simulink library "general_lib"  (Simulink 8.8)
settings: Solver=ode45  StartTime=0.0  StopTime=10.0  RelTol=1e-3  EnableMultiTasking=on
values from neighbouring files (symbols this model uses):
  transmission = class_transmission_data    [class_test_data.m]
undefined symbols (not defined in the file or in its folder): AxisNumber, BreakpointData, BreakpointsForDimension1, BreakpointsForDimension2, BreakpointsForDimension3, DelayTimeSecs, down_time, ExtrapolateAbove, ExtrapolateBelow, InitialCondition, InitialValue, LookupStructure, MaximumIndicesForEachDimension, MultiplyPosInputs, Normalize, NumPhases, struct_var, Table, test_mat, up_time, UpperSaturationLimit, VerboseLevel, VerboseSignal
libraries: general_lib x5, simulink x3

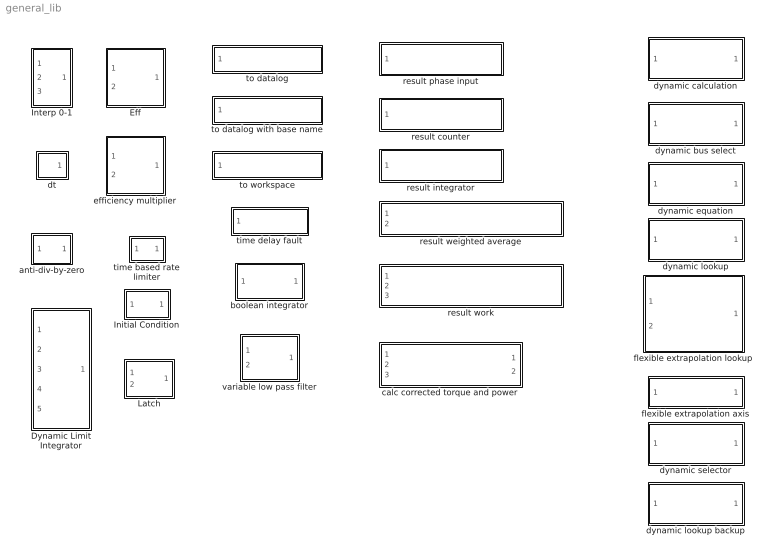
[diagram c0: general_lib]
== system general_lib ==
  Dynamic Limit Integrator : Subsystem
  Eff : Subsystem
  Initial Condition : Subsystem
  Interp 0-1 : Subsystem
  Latch : Subsystem
  anti-div-by-zero : Subsystem
  boolean integrator : Subsystem
  calc corrected torque and power : Subsystem
  dt : Subsystem
  dynamic bus select : Subsystem
  dynamic calculation : Subsystem
  dynamic equation : Subsystem
  dynamic lookup : Subsystem
  dynamic lookup backup : Subsystem  Commented=on
  dynamic selector : Subsystem  BlockChoice=dynamic equation
  efficiency multiplier : Subsystem
  flexible extrapolation axis : Subsystem
  flexible extrapolation lookup : Subsystem
  result counter : Subsystem
  result integrator : Subsystem
  result phase input : Subsystem
  result weighted average : Subsystem
  result work : Subsystem
  time based rate limiter : Subsystem
  time delay fault : Subsystem
  to datalog : Subsystem
  to datalog with base name : Subsystem
  to workspace : Subsystem
  variable low pass filter : Subsystem

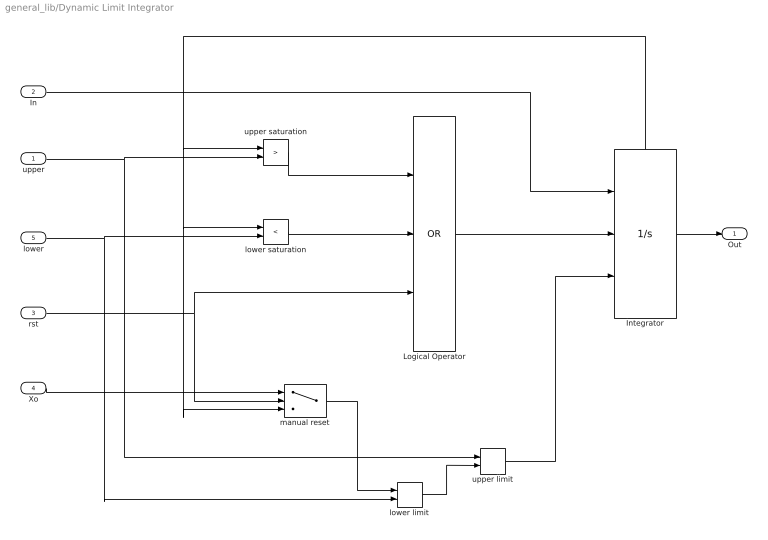
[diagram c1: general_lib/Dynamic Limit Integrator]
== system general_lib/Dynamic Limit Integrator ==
  upper : Inport
  In : Inport  Port=2
  rst : Inport  Port=3
  Xo : Inport  Port=4
  lower : Inport  Port=5
  Integrator : Integrator  ExternalReset=level  InitialConditionSource=external  ShowStatePort=on
  Logical Operator : Logic  Operator=OR  Inputs=3  AllPortsSameDT=off  OutDataTypeStr=boolean
  lower limit : MinMax  Function=max  Inputs=2  ZeroCross=off
  lower saturation : RelationalOperator  Operator=<  OutDataTypeStr=boolean
  manual reset : Switch  Criteria=u2 ~= 0
  upper limit : MinMax  Inputs=2
  upper saturation : RelationalOperator  Operator=>  OutDataTypeStr=boolean
  Out : Outport
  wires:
  Integrator/State -> manual reset/3, lower saturation/1, upper saturation/1
  Integrator/1 -> Out/1
  lower limit/1 -> upper limit/2
  Xo/1 -> manual reset/1
  rst/1 -> manual reset/2, Logical Operator/3
  upper saturation/1 -> Logical Operator/1
  lower saturation/1 -> Logical Operator/2
  Logical Operator/1 -> Integrator/2
  In/1 -> Integrator/1
  lower/1 -> lower limit/2, lower saturation/2
  upper limit/1 -> Integrator/3
  upper/1 -> upper saturation/2, upper limit/1
  manual reset/1 -> lower limit/1

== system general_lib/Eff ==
  Efficiency : Inport
  Input : Inport  Port=2
  Math Function : Math  Operator=reciprocal
  Product1 : Product
  Switch : Switch  ZeroCross=off
  Output : Outport
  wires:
  Switch/1 -> Product1/1
  Efficiency/1 -> Math Function/1, Switch/1
  Input/1 -> Switch/2, Product1/2
  Product1/1 -> Output/1
  Math Function/1 -> Switch/3

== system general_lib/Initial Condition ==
  In : Inport
  Constant2 : Constant
  IC Switch : Switch  Criteria=u2 ~= 0
  IC Value : Constant  Value=InitialValue
  Memory : Memory
  Out : Outport
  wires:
  IC Switch/1 -> Out/1
  In/1 -> IC Switch/1
  IC Value/1 -> IC Switch/3
  Memory/1 -> IC Switch/2
  Constant2/1 -> Memory/1

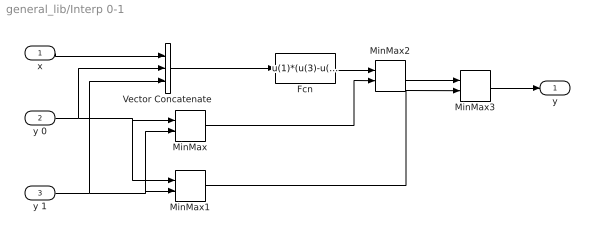
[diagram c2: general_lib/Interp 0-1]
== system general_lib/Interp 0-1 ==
  x : Inport
  y 0 : Inport  Port=2
  y 1 : Inport  Port=3
  Fcn : Fcn  Expr=u(1)*(u(3)-u(2)) + u(2)
  MinMax : MinMax  Inputs=2  ZeroCross=off
  MinMax1 : MinMax  Function=max  Inputs=2  ZeroCross=off
  MinMax2 : MinMax  Function=max  Inputs=2  ZeroCross=off
  MinMax3 : MinMax  Inputs=2  ZeroCross=off
  Vector Concatenate : Concatenate  NumInputs=3
  y : Outport
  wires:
  y 0/1 -> Vector Concatenate/2, MinMax1/1, MinMax/1
  Vector Concatenate/1 -> Fcn/1
  y 1/1 -> Vector Concatenate/3, MinMax/2, MinMax1/2
  MinMax3/1 -> y/1
  x/1 -> Vector Concatenate/1
  MinMax/1 -> MinMax2/2
  MinMax1/1 -> MinMax3/2
  MinMax2/1 -> MinMax3/1
  Fcn/1 -> MinMax2/1

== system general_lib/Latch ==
  On : Inport  PortDimensions=1
  Off : Inport  Port=2  PortDimensions=1
  Combinatorial  Logic : CombinatorialLogic  TruthTable=[0;1;0;0;1;1;(tb==2);(tb>=2)]
  Memory2 : Memory  X0=InitialCondition
  Mux : Mux  Inputs=3
  State : Outport  PortDimensions=1
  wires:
  Combinatorial  Logic/1 -> Memory2/1, State/1
  Mux/1 -> Combinatorial  Logic/1
  Memory2/1 -> Mux/3
  On/1 -> Mux/1
  Off/1 -> Mux/2

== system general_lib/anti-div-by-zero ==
  note: force sign(0) = 1, not 0!
  In : Inport
  Abs : Abs  ZeroCross=off
  Constant : Constant  Value=eps
  MinMax : MinMax  Function=max  Inputs=2  ZeroCross=off
  Product2 : Product
  Relay : Relay  OnSwitchValue=-eps  OffSwitchValue=-eps  OffOutputValue=-1  ZeroCross=off
  Out : Outport
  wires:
  Product2/1 -> Out/1
  In/1 -> Relay/1, Abs/1
  Abs/1 -> MinMax/1
  MinMax/1 -> Product2/1
  Constant/1 -> MinMax/2
  Relay/1 -> Product2/2

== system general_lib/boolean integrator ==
  bool : Inport
  Constant : Constant  Value=Normalize
  Data Type Conversion2 : DataTypeConversion  OutDataTypeStr=double
  Integrator1 : Integrator  ExternalReset=falling  LimitOutput=on  UpperSaturationLimit=UpperSaturationLimit  LowerSaturationLimit=0
  Switch : Switch  Criteria=u2 > Threshold
  normalize : Gain  Gain=1/UpperSaturationLimit
  out : Outport
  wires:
  Data Type Conversion2/1 -> Integrator1/2, Integrator1/1
  bool/1 -> Data Type Conversion2/1
  Constant/1 -> Switch/2
  Integrator1/1 -> normalize/1, Switch/3
  normalize/1 -> Switch/1
  Switch/1 -> out/1

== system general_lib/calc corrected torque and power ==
  trq_Nm : Inport
  spd_radps : Inport  Port=2
  upstream_iner_kgm2 : Inport  Port=3
  Derivative : Derivative  CoefficientInTFapproximation=1e6
  Product1 : Product
  Product2 : Product
  Subtract : Sum  Inputs=+-
  corr_trq_Nm : Outport
  corr_pwr_W : Outport  Port=2
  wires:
  trq_Nm/1 -> Subtract/1
  Subtract/1 -> Product2/1, corr_trq_Nm/1
  upstream_iner_kgm2/1 -> Product1/2
  spd_radps/1 -> Product2/2, Derivative/1
  Derivative/1 -> Product1/1
  Product1/1 -> Subtract/2
  Product2/1 -> corr_pwr_W/1

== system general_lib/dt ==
  Clock : Clock
  Memory1 : Memory
  Sum : Sum  Inputs=|-+
  dt : Outport
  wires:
  Sum/1 -> dt/1
  Memory1/1 -> Sum/1
  Clock/1 -> Memory1/1, Sum/2

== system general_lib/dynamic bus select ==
  bus : Inport
  Bus Selector : BusSelector  OutputSignals=signal1,bus.signal2  OutputAsBus=on
  Reshape : Reshape
  out : Outport
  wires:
  Reshape/1 -> out/1
  bus/1 -> Bus Selector/1
  Bus Selector/1 -> Reshape/1

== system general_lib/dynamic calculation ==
  bus : Inport
  dynamic selector : Subsystem  BlockChoice=dynamic equation
  out : Outport
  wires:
  bus/1 -> dynamic selector/1(bus)
  dynamic selector/1(out) -> out/1

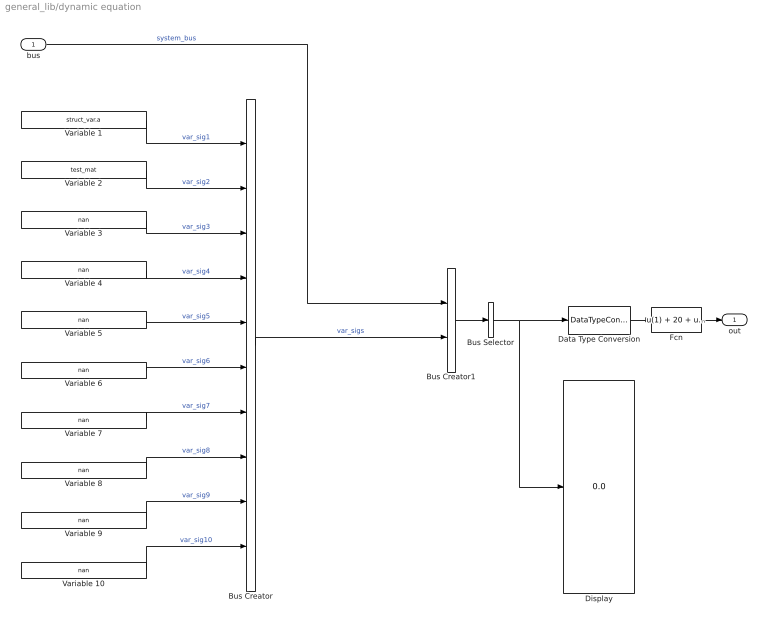
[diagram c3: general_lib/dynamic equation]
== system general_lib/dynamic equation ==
  bus : Inport
  Bus Creator : BusCreator  Inputs=10
  Bus Creator1 : BusCreator  Inputs=2
  Bus Selector : BusSelector  OutputSignals=sig_1,var_sigs.var_sig1,var_sigs.var_sig2  OutputAsBus=on
  Data Type Conversion : DataTypeConversion  OutDataTypeStr=double
  Display : Display
  Fcn : Fcn  Expr=u(1) + 20 + u(3) + u(2)
  Variable 1 : Constant  Value=struct_var.a
  Variable {3..10} (8 alike) : Constant  Value=nan
  Variable 2 : Constant  Value=test_mat
  out : Outport
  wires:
  Variable 10/1 -> Bus Creator/10  "var_sig10"
  Variable 9/1 -> Bus Creator/9  "var_sig9"
  Variable 8/1 -> Bus Creator/8  "var_sig8"
  Variable 7/1 -> Bus Creator/7  "var_sig7"
  Variable 6/1 -> Bus Creator/6  "var_sig6"
  Variable 5/1 -> Bus Creator/5  "var_sig5"
  Variable 4/1 -> Bus Creator/4  "var_sig4"
  Variable 3/1 -> Bus Creator/3  "var_sig3"
  Variable 2/1 -> Bus Creator/2  "var_sig2"
  Variable 1/1 -> Bus Creator/1  "var_sig1"
  Bus Creator/1 -> Bus Creator1/2  "var_sigs"
  bus/1 -> Bus Creator1/1  "system_bus"
  Fcn/1 -> out/1
  Bus Creator1/1 -> Bus Selector/1
  Bus Selector/1 -> Display/1, Data Type Conversion/1
  Data Type Conversion/1 -> Fcn/1

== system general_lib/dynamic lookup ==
  bus : Inport
  Bus Selector : BusSelector  OutputSignals=gb.gb_cmd_gear,gb_spd_in_radps,ctrl.gb_line_press_bar
  Lookup : Lookup_n-D  NumberOfTableDimensions=10  BreakpointsForDimension1=LookupStructure.axis_1.breakpoints  BreakpointsForDimension2=LookupStructure.axis_2.breakpoints  BreakpointsForDimension3=LookupStructure.axis_3.breakpoints  BreakpointsForDimension4=LookupStructure.axis_4.breakpoints  BreakpointsForDimension5=LookupStructure.axis_5.breakpoints  BreakpointsForDimension6=LookupStructure.axis_6.breakpoints  BreakpointsForDimension7=LookupStructure.axis_7.breakpoints  BreakpointsForDimension8=LookupStructure.axis_8.breakpoints  BreakpointsForDimension9=LookupStructure.axis_9.breakpoints  BreakpointsForDimension10=LookupStructure.axis_10.breakpoints  IndexSearchMethod=Linear search  BeginIndexSearchUsingPreviousIndexResult=on  Table=LookupStructure.table  DiagnosticForOutOfRangeInput=Warning  InternalRulePriority=Speed  RndMeth=Simplest  SupportTunableTableSize=on  MaximumIndicesForEachDimension=LookupStructure.table_size
  out : Outport
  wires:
  Lookup/1 -> out/1
  bus/1 -> Bus Selector/1

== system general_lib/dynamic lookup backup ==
  bus : Inport
  Bus Selector : BusSelector  OutputSignals=gb.gb_cmd_gear,gb_spd_in_radps,ctrl.gb_line_press_bar
  Lookup : Lookup_n-D  NumberOfTableDimensions=10  BreakpointsForDimension1=LookupStructure.axis_1.breakpoints  BreakpointsForDimension2=LookupStructure.axis_2.breakpoints  BreakpointsForDimension3=LookupStructure.axis_3.breakpoints  BreakpointsForDimension4=LookupStructure.axis_4.breakpoints  BreakpointsForDimension5=LookupStructure.axis_5.breakpoints  BreakpointsForDimension6=LookupStructure.axis_6.breakpoints  BreakpointsForDimension7=LookupStructure.axis_7.breakpoints  BreakpointsForDimension8=LookupStructure.axis_7.breakpoints  BreakpointsForDimension9=LookupStructure.axis_7.breakpoints  BreakpointsForDimension10=LookupStructure.axis_7.breakpoints  IndexSearchMethod=Linear search  BeginIndexSearchUsingPreviousIndexResult=on  Table=LookupStructure.table  ExtrapMethod=Clip  DiagnosticForOutOfRangeInput=Warning  InternalRulePriority=Speed  RndMeth=Simplest  MaximumIndicesForEachDimension=MaximumIndicesForEachDimension
  out : Outport
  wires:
  Lookup/1 -> out/1
  bus/1 -> Bus Selector/1

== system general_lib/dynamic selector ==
  bus : Inport
  dynamic equation : general_lib/dynamic equation  DynamicExpression='@sig_1 + 20 + test_mat + struct_var.a '  DynamicExpressionEval=@sig_1 + 20 + test_mat + struct_var.a
  out : Outport
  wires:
  bus/1 -> dynamic equation/1
  dynamic equation/1 -> out/1

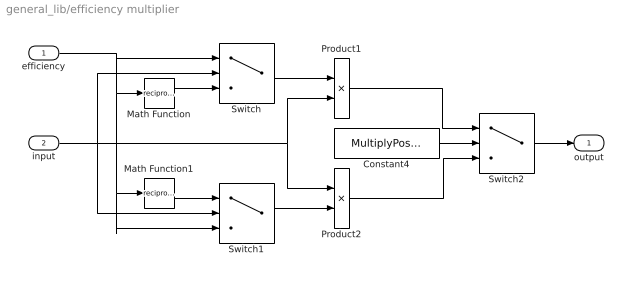
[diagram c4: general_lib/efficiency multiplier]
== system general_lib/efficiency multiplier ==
  efficiency : Inport
  input : Inport  Port=2
  Constant4 : Constant  Value=MultiplyPosInputs
  Math Function : Math  Operator=reciprocal
  Math Function1 : Math  Operator=reciprocal
  Product1 : Product
  Product2 : Product
  Switch : Switch  ZeroCross=off
  Switch1 : Switch  ZeroCross=off
  Switch2 : Switch  Criteria=u2 > Threshold  ZeroCross=off
  output : Outport
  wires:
  Switch/1 -> Product1/1
  Math Function/1 -> Switch/3
  Switch1/1 -> Product2/2
  efficiency/1 -> Switch1/3, Math Function1/1, Math Function/1, Switch/1
  input/1 -> Switch/2, Product1/2, Product2/1, Switch1/2
  Math Function1/1 -> Switch1/1
  Switch2/1 -> output/1
  Product1/1 -> Switch2/1
  Product2/1 -> Switch2/3
  Constant4/1 -> Switch2/2

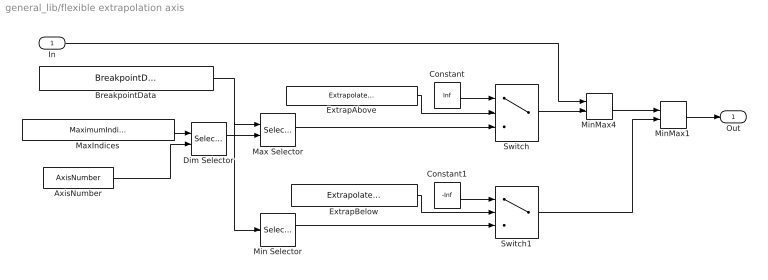
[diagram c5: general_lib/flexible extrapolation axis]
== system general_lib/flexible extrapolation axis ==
  In : Inport
  AxisNumber : Constant  Value=AxisNumber
  BreakpointData : Constant  Value=BreakpointData
  Constant : Constant  Value=Inf
  Constant1 : Constant  Value=-Inf
  Dim Selector : Selector  IndexOptions=Index vector (port)  Indices=BreakpointLength  OutputSizes=1
  ExtrapAbove : Constant  Value=ExtrapolateAbove
  ExtrapBelow : Constant  Value=ExtrapolateBelow
  Max Selector : Selector  IndexMode=Zero-based  IndexOptions=Index vector (port)  Indices=BreakpointLength  OutputSizes=1
  MaxIndices : Constant  Value=MaximumIndicesForEachDimension
  Min Selector : Selector  IndexMode=Zero-based  IndexOptions=Index vector (dialog)  Indices=0  OutputSizes=1
  MinMax1 : MinMax  Function=max  Inputs=2  ZeroCross=off
  MinMax4 : MinMax  Inputs=2  ZeroCross=off
  Switch : Switch  Criteria=u2 ~= 0  ZeroCross=off
  Switch1 : Switch  Criteria=u2 ~= 0  ZeroCross=off
  Out : Outport
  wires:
  MinMax1/1 -> Out/1
  MinMax4/1 -> MinMax1/1
  In/1 -> MinMax4/1
  Switch1/1 -> MinMax1/2
  Switch/1 -> MinMax4/2
  Max Selector/1 -> Switch/3
  ExtrapAbove/1 -> Switch/2
  ExtrapBelow/1 -> Switch1/2
  Min Selector/1 -> Switch1/3
  Constant1/1 -> Switch1/1
  Constant/1 -> Switch/1
  BreakpointData/1 -> Min Selector/1, Max Selector/1
  MaxIndices/1 -> Dim Selector/1
  AxisNumber/1 -> Dim Selector/2
  Dim Selector/1 -> Max Selector/2

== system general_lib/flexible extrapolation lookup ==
  In1 : Inport
  In2 : Inport  Port=2
  Lookup : Lookup_n-D  BreakpointsForDimension1=BreakpointsForDimension1  BreakpointsForDimension2=BreakpointsForDimension2  BreakpointsForDimension3=BreakpointsForDimension3  BreakpointsForDimension4=BreakpointsForDimension4  BreakpointsForDimension5=BreakpointsForDimension5  BreakpointsForDimension6=BreakpointsForDimension6  BreakpointsForDimension7=BreakpointsForDimension7  BreakpointsForDimension8=BreakpointsForDimension8  BreakpointsForDimension9=BreakpointsForDimension9  BreakpointsForDimension10=BreakpointsForDimension10  IndexSearchMethod=Linear search  BeginIndexSearchUsingPreviousIndexResult=on  Table=Table  InternalRulePriority=Speed  RndMeth=Simplest  MaximumIndicesForEachDimension=MaximumIndicesForEachDimension
  axis1 : general_lib/flexible extrapolation axis  BreakpointData=BreakpointsForDimension1  ExtrapolateAbove=ExtrapolateAboveDimension1  ExtrapolateBelow=ExtrapolateBelowDimension1  MaximumIndicesForEachDimension=MaximumIndicesForEachDimension  AxisNumber=1
  axis2 : general_lib/flexible extrapolation axis  BreakpointData=BreakpointsForDimension2  ExtrapolateAbove=ExtrapolateAboveDimension2  ExtrapolateBelow=ExtrapolateBelowDimension2  MaximumIndicesForEachDimension=MaximumIndicesForEachDimension  AxisNumber=2
  Out : Outport
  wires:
  axis1/1 -> Lookup/1
  In1/1 -> axis1/1
  axis2/1 -> Lookup/2
  In2/1 -> axis2/1
  Lookup/1 -> Out/1

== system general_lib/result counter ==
  in : Inport
  Data Type Conversion : DataTypeConversion  OutDataTypeStr=double
  Phase Memory : Memory
  Phase To Workspace : ToWorkspace  VariableName=result__phase_counts  SampleTime=-1
  Product : Product
  Sum : Sum  Inputs=|++
  Sum1 : Sum  Inputs=|++
  Total Memory : Memory
  Total To Workspace : ToWorkspace  VariableName=result__total_counts  SampleTime=-1
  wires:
  Phase Memory/1 -> Sum/2, Phase To Workspace/1
  [REVS_phase_flag] -> Product/1
  Product/1 -> Sum/1
  Total Memory/1 -> Total To Workspace/1, Sum1/2
  in/1 -> Data Type Conversion/1
  Sum/1 -> Phase Memory/1
  Sum1/1 -> Total Memory/1
  Data Type Conversion/1 -> Sum1/1, Product/2

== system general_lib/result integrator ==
  in : Inport
  Data Type Conversion : DataTypeConversion  OutDataTypeStr=double
  Integrator1 : Integrator  UpperSaturationLimit=Inf  LowerSaturationLimit=0  ZeroCross=off
  Integrator2 : Integrator  UpperSaturationLimit=Inf  LowerSaturationLimit=0  ZeroCross=off
  Phase To Workspace : ToWorkspace  VariableName=result__phase_distance_m  SampleTime=-1
  Product1 : Product  Multiplication=Matrix(*)
  Reshape : Reshape
  Total To Workspace : ToWorkspace  VariableName=result__total_distance_m  SampleTime=-1
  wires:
  in/1 -> Data Type Conversion/1
  Integrator1/1 -> Total To Workspace/1
  Product1/1 -> Integrator2/1
  [REVS_phase_flag] -> Product1/2
  Integrator2/1 -> Phase To Workspace/1
  Data Type Conversion/1 -> Reshape/1
  Reshape/1 -> Product1/1, Integrator1/1

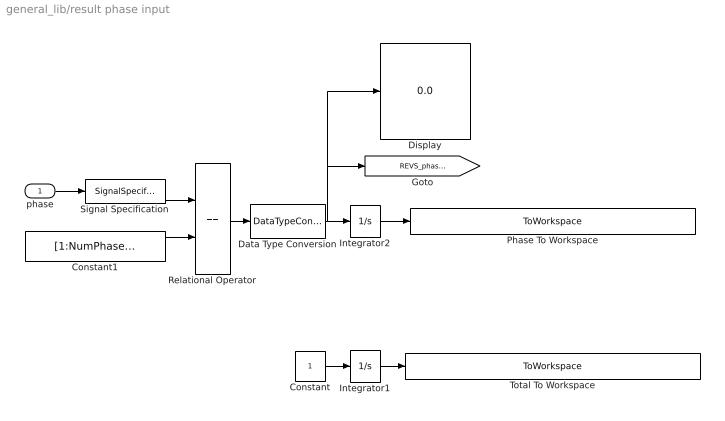
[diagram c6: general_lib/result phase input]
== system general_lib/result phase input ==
  phase : Inport
  Constant : Constant
  Constant1 : Constant  Value=[1:NumPhases]  VectorParams1D=off
  Data Type Conversion : DataTypeConversion
  Display : Display
  Integrator1 : Integrator  UpperSaturationLimit=Inf  LowerSaturationLimit=0  ZeroCross=off
  Integrator2 : Integrator  UpperSaturationLimit=Inf  LowerSaturationLimit=0  ZeroCross=off
  Phase To Workspace : ToWorkspace  VariableName=result__phase_distance_m  SampleTime=-1
  Relational Operator : RelationalOperator  Operator===  OutDataTypeStr=boolean  ZeroCross=off
  Signal Specification : SignalSpecification  Dimensions=1
  Total To Workspace : ToWorkspace  VariableName=result__total_distance_m  SampleTime=-1
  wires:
  Integrator2/1 -> Phase To Workspace/1
  Relational Operator/1 -> Data Type Conversion/1
  Integrator1/1 -> Total To Workspace/1
  Constant/1 -> Integrator1/1
  Constant1/1 -> Relational Operator/2
  phase/1 -> Signal Specification/1
  Data Type Conversion/1 -> Display/1, [REVS_phase_flag], Integrator2/1
  Signal Specification/1 -> Relational Operator/1

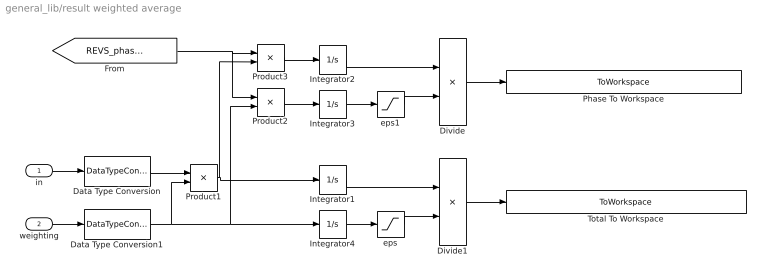
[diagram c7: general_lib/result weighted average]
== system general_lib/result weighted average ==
  in : Inport
  weighting : Inport  Port=2
  Data Type Conversion : DataTypeConversion  OutDataTypeStr=double
  Data Type Conversion1 : DataTypeConversion  OutDataTypeStr=double
  Divide : Product  Inputs=*/
  Divide1 : Product  Inputs=*/
  Integrator{1..4} (4 alike) : Integrator  UpperSaturationLimit=Inf  LowerSaturationLimit=0  ZeroCross=off
  Phase To Workspace : ToWorkspace  VariableName=result__phase_avg_speed_radps  SampleTime=-1
  Product1 : Product
  Product2 : Product
  Product3 : Product
  Total To Workspace : ToWorkspace  VariableName=result__total_avg_speed_radps  SampleTime=-1
  eps : Saturate  UpperLimit=inf  LowerLimit=eps
  eps1 : Saturate  UpperLimit=inf  LowerLimit=eps
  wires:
  Integrator2/1 -> Divide/1
  [REVS_phase_flag] -> Product3/1, Product2/1
  Product3/1 -> Integrator2/1
  Integrator1/1 -> Divide1/1
  in/1 -> Data Type Conversion/1
  weighting/1 -> Data Type Conversion1/1
  Data Type Conversion1/1 -> Product2/2, Integrator4/1, Product1/2
  Product2/1 -> Integrator3/1
  Product1/1 -> Product3/2, Integrator1/1
  Integrator4/1 -> eps/1
  Integrator3/1 -> eps1/1
  Divide/1 -> Phase To Workspace/1
  Divide1/1 -> Total To Workspace/1
  eps/1 -> Divide1/2
  eps1/1 -> Divide/2
  Data Type Conversion/1 -> Product1/1

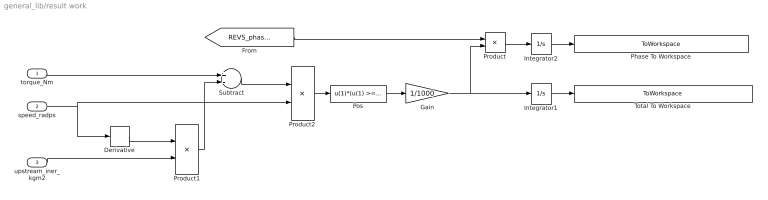
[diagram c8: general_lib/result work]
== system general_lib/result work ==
  torque_Nm : Inport
  speed_radps : Inport  Port=2
  upstream_iner_kgm2 : Inport  Port=3
  Derivative : Derivative  CoefficientInTFapproximation=1e6
  Gain : Gain  Gain=1/1000
  Integrator1 : Integrator  UpperSaturationLimit=Inf  LowerSaturationLimit=0  ZeroCross=off
  Integrator2 : Integrator  UpperSaturationLimit=Inf  LowerSaturationLimit=0  ZeroCross=off
  Phase To Workspace : ToWorkspace  VariableName=result__phase_distance_m  SampleTime=-1
  Pos : Fcn  Expr=u(1)*(u(1) >= 0)
  Product : Product
  Product1 : Product
  Product2 : Product
  Subtract : Sum  Inputs=+-
  Total To Workspace : ToWorkspace  VariableName=result__total_distance_m  SampleTime=-1
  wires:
  torque_Nm/1 -> Subtract/1
  Integrator1/1 -> Total To Workspace/1
  Product/1 -> Integrator2/1
  [REVS_phase_flag] -> Product/1
  Integrator2/1 -> Phase To Workspace/1
  Subtract/1 -> Product2/1
  upstream_iner_kgm2/1 -> Product1/2
  speed_radps/1 -> Product2/2, Derivative/1
  Derivative/1 -> Product1/1
  Product1/1 -> Subtract/2
  Gain/1 -> Product/2, Integrator1/1
  Pos/1 -> Gain/1
  Product2/1 -> Pos/1

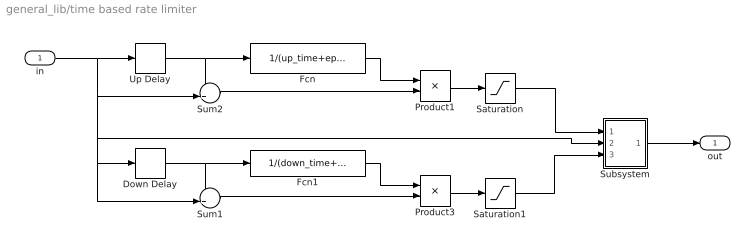
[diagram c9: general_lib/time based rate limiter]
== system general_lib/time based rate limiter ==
  in : Inport
  Down Delay : TransportDelay  DelayTime=max(eps, down_time)  BufferSize=10240  TransDelayFeedthrough=on
  Fcn : Fcn  Expr=1/(up_time+eps)
  Fcn1 : Fcn  Expr=1/(down_time+eps)
  Product1 : Product
  Product3 : Product
  Saturation : Saturate  UpperLimit=Inf  LowerLimit=0
  Saturation1 : Saturate  UpperLimit=0  LowerLimit=-Inf
  Subsystem : Subsystem
  Sum1 : Sum  Inputs=-+|
  Sum2 : Sum  Inputs=-+|
  Up Delay : TransportDelay  DelayTime=max(eps, up_time)  TransDelayFeedthrough=on
  out : Outport
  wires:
  Subsystem/1(Y) -> out/1
  Fcn1/1 -> Product3/1
  Fcn/1 -> Product1/1
  Up Delay/1 -> Sum2/1, Fcn/1
  Down Delay/1 -> Sum1/1, Fcn1/1
  Sum1/1 -> Product3/2
  Product3/1 -> Saturation1/1
  Product1/1 -> Saturation/1
  Saturation/1 -> Subsystem/1(up)
  Saturation1/1 -> Subsystem/3(lo)
  Sum2/1 -> Product1/2
  in/1 -> Up Delay/1, Sum2/2, Down Delay/1, Sum1/2, Subsystem/2(u)

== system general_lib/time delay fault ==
  " condition" : Inport
  Assertion : Assertion  AssertionFailFcn=error('There Was An Error')
  Compare To Constant1 : simulink/Logic and Bit Operations/Compare To Constant  relop=<  const=DelayTimeSecs  OutDataTypeStr=boolean  ZeroCross=off
  Compare To Constant2 : simulink/Logic and Bit Operations/Compare To Constant  relop=>  const=DelayTimeSecs + 0.1  OutDataTypeStr=boolean  ZeroCross=off
  Data Type Conversion : DataTypeConversion
  Integrator1 : Integrator  ExternalReset=falling  ZeroCross=off
  Stop Simulation : Stop
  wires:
  Compare To Constant1/1 -> Assertion/1
  " condition"/1 -> Data Type Conversion/1
  Integrator1/1 -> Compare To Constant2/1, Compare To Constant1/1
  Data Type Conversion/1 -> Integrator1/2, Integrator1/1
  Compare To Constant2/1 -> Stop Simulation/1

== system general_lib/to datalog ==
  Var : Inport
  Constant : Constant  Value=VerboseSignal
  Constant1 : Constant  Value=VerboseLevel
  Relational Operator : RelationalOperator  OutDataTypeStr=boolean  ZeroCross=off
  Subsystem : Subsystem
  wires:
  Var/1 -> Subsystem/1(In1)
  Relational Operator/1 -> Subsystem/Enable
  Constant/1 -> Relational Operator/1
  Constant1/1 -> Relational Operator/2

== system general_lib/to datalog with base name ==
  Var : Inport
  Constant : Constant  Value=VerboseSignal
  Constant1 : Constant  Value=VerboseLevel
  Relational Operator : RelationalOperator  OutDataTypeStr=boolean  ZeroCross=off
  Subsystem : Subsystem
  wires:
  Var/1 -> Subsystem/1(Var)
  Constant/1 -> Relational Operator/1
  Relational Operator/1 -> Subsystem/Enable
  Constant1/1 -> Relational Operator/2

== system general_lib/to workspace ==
  Var : Inport
  Constant : Constant  Value=VerboseSignal
  Constant1 : Constant  Value=VerboseLevel
  Relational Operator : RelationalOperator  OutDataTypeStr=boolean  ZeroCross=off
  Subsystem : Subsystem
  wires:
  Var/1 -> Subsystem/1(In1)
  Relational Operator/1 -> Subsystem/Enable
  Constant/1 -> Relational Operator/1
  Constant1/1 -> Relational Operator/2

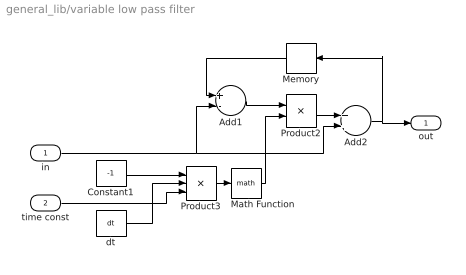
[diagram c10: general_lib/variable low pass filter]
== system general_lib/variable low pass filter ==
  in : Inport
  time const : Inport  Port=2
  Add1 : Sum  Inputs=+-
  Add2 : Sum
  Constant1 : Constant  Value=-1
  Math Function : Math
  Memory : Memory  X0=max(transmission.gear.ratio)
  Product2 : Product
  Product3 : Product  Inputs=**/
  dt : general_lib/dt
  out : Outport
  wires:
  dt/1 -> Product3/2
  Add2/1 -> out/1, Memory/1
  Memory/1 -> Add1/1
  Add1/1 -> Product2/1
  Product2/1 -> Add2/1
  Math Function/1 -> Product2/2
  Constant1/1 -> Product3/1
  Product3/1 -> Math Function/1
  in/1 -> Add2/2, Add1/2
  time const/1 -> Product3/3

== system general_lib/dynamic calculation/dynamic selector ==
  bus : Inport
  dynamic equation : general_lib/dynamic equation  DynamicExpression=DynamicCalculation.function
  out : Outport
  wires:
  bus/1 -> dynamic equation/1
  dynamic equation/1 -> out/1

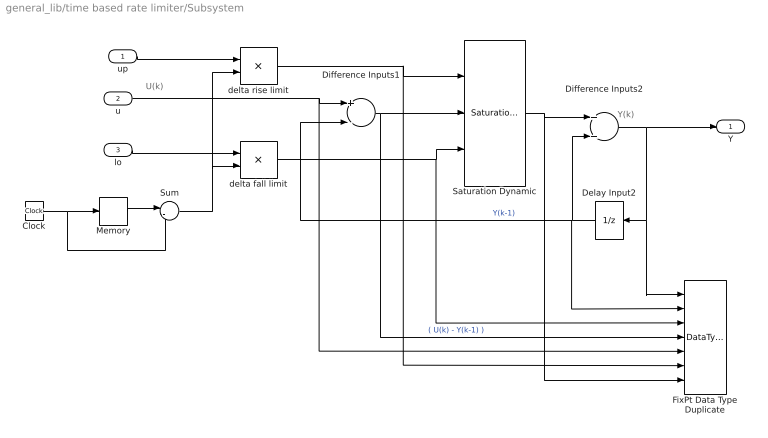
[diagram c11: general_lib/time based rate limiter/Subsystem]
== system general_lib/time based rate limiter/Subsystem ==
  note: Y(k)
  note: U(k)
  up : Inport
  u : Inport  Port=2
  lo : Inport  Port=3
  Clock : Clock
  Delay Input2 : UnitDelay  Description=Store in Global RAM  DisableCoverage=on  SampleTime=-1
  Difference Inputs1 : Sum  Description=Add in CPU  DisableCoverage=on  Inputs=+-  OutDataTypeStr=Inherit: Inherit via back propagation
  Difference Inputs2 : Sum  Description=Add in CPU  OutDataTypeStr=Inherit: Inherit via back propagation
  FixPt Data Type Duplicate : DataTypeDuplicate  DisableCoverage=on  NumInputPorts=7
  Memory : Memory
  Saturation Dynamic : simulink/Discontinuities/Saturation Dynamic  OutMin=[]  OutMax=[]  OutDataTypeStr=Inherit: Same as second input  OutDataType=fixdt(1, 16)  OutScaling=2^-10  DoSatur=off
  Sum : Sum  Inputs=|-+
  delta fall limit : Product  DisableCoverage=on  Inputs=**  OutDataTypeStr=Inherit: Inherit via back propagation
  delta rise limit : Product  DisableCoverage=on  Inputs=**  OutDataTypeStr=Inherit: Inherit via back propagation
  Y : Outport  InitialOutput=0
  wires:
  Clock/1 -> Memory/1, Sum/2
  Memory/1 -> Sum/1
  delta fall limit/1 -> FixPt Data Type Duplicate/3, Saturation Dynamic/3
  lo/1 -> delta fall limit/1
  Difference Inputs2/1 -> Delay Input2/1, FixPt Data Type Duplicate/1, Y/1
  Sum/1 -> delta fall limit/2, delta rise limit/2
  u/1 -> Difference Inputs1/1, FixPt Data Type Duplicate/5
  delta rise limit/1 -> FixPt Data Type Duplicate/6, Saturation Dynamic/1
  Delay Input2/1 -> Difference Inputs1/2, FixPt Data Type Duplicate/2, Difference Inputs2/2  "Y(k-1)"
  Saturation Dynamic/1 -> Difference Inputs2/1, FixPt Data Type Duplicate/7
  up/1 -> delta rise limit/1
  Difference Inputs1/1 -> FixPt Data Type Duplicate/4, Saturation Dynamic/2  "( U(k) - Y(k-1) )"

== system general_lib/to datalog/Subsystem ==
  In1 : Inport
  Enable : EnablePort
  To Workspace : ToWorkspace  VariableName=datalog__struct__var  SampleTime=-1
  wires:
  In1/1 -> To Workspace/1

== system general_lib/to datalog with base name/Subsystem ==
  Var : Inport
  Enable : EnablePort
  To Workspace : ToWorkspace  VariableName=datalog__struct__var  SampleTime=-1
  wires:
  Var/1 -> To Workspace/1

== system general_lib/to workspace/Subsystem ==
  In1 : Inport
  Enable : EnablePort
  To Workspace : ToWorkspace  VariableName=struct__var  SampleTime=-1
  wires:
  In1/1 -> To Workspace/1
